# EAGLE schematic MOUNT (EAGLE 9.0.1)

## Sheet 1 of 2: Board to Board Headers
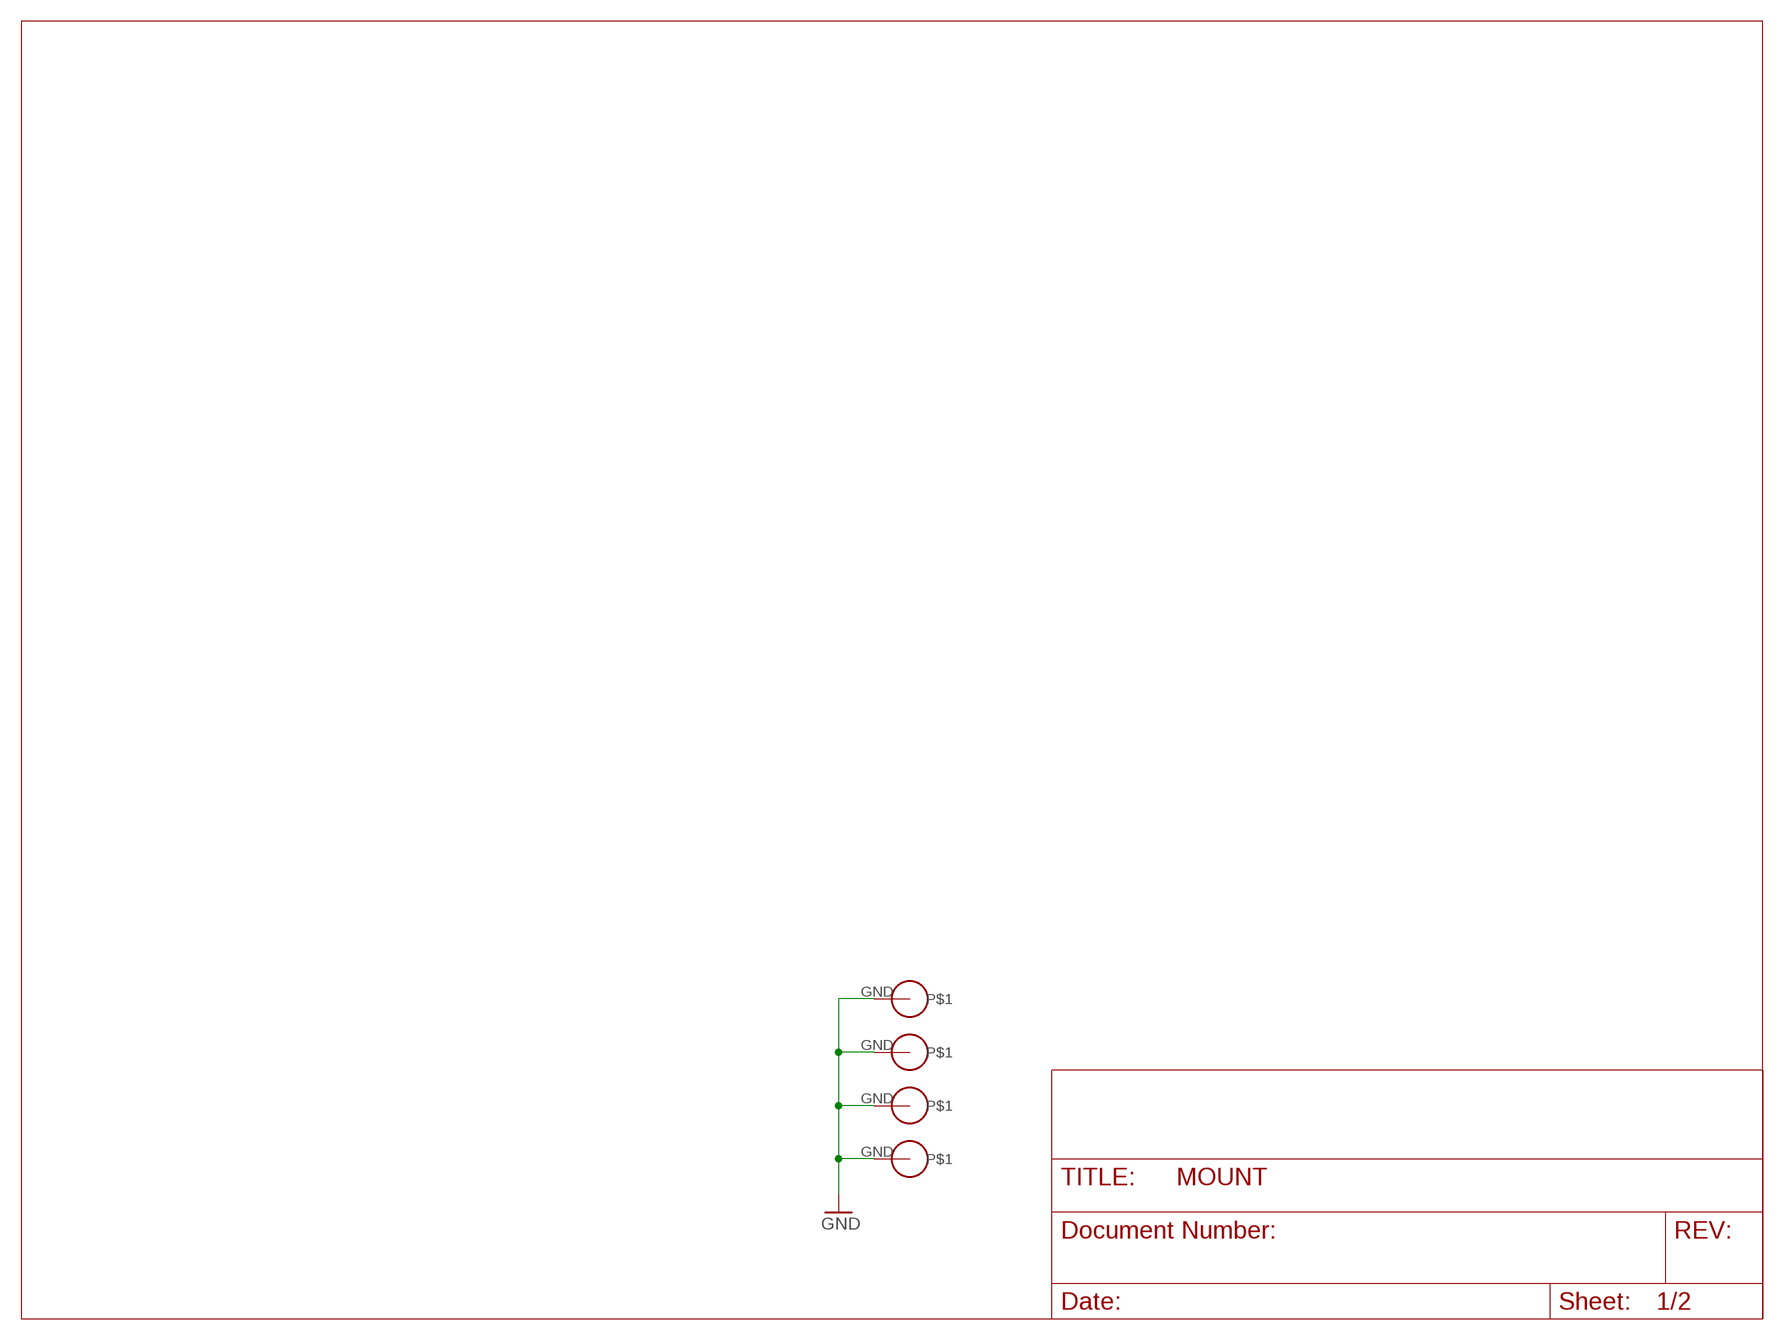
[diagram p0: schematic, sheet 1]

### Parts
U$1  PS/104-MOUNTING-HOLE  [PC/104-MOUNTING-HOLE]
U$2  PS/104-MOUNTING-HOLE  [PC/104-MOUNTING-HOLE]
U$3  PS/104-MOUNTING-HOLE  [PC/104-MOUNTING-HOLE]
U$4  PS/104-MOUNTING-HOLE  [PC/104-MOUNTING-HOLE]

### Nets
GND: U$1.GND U$2.GND U$3.GND U$4.GND

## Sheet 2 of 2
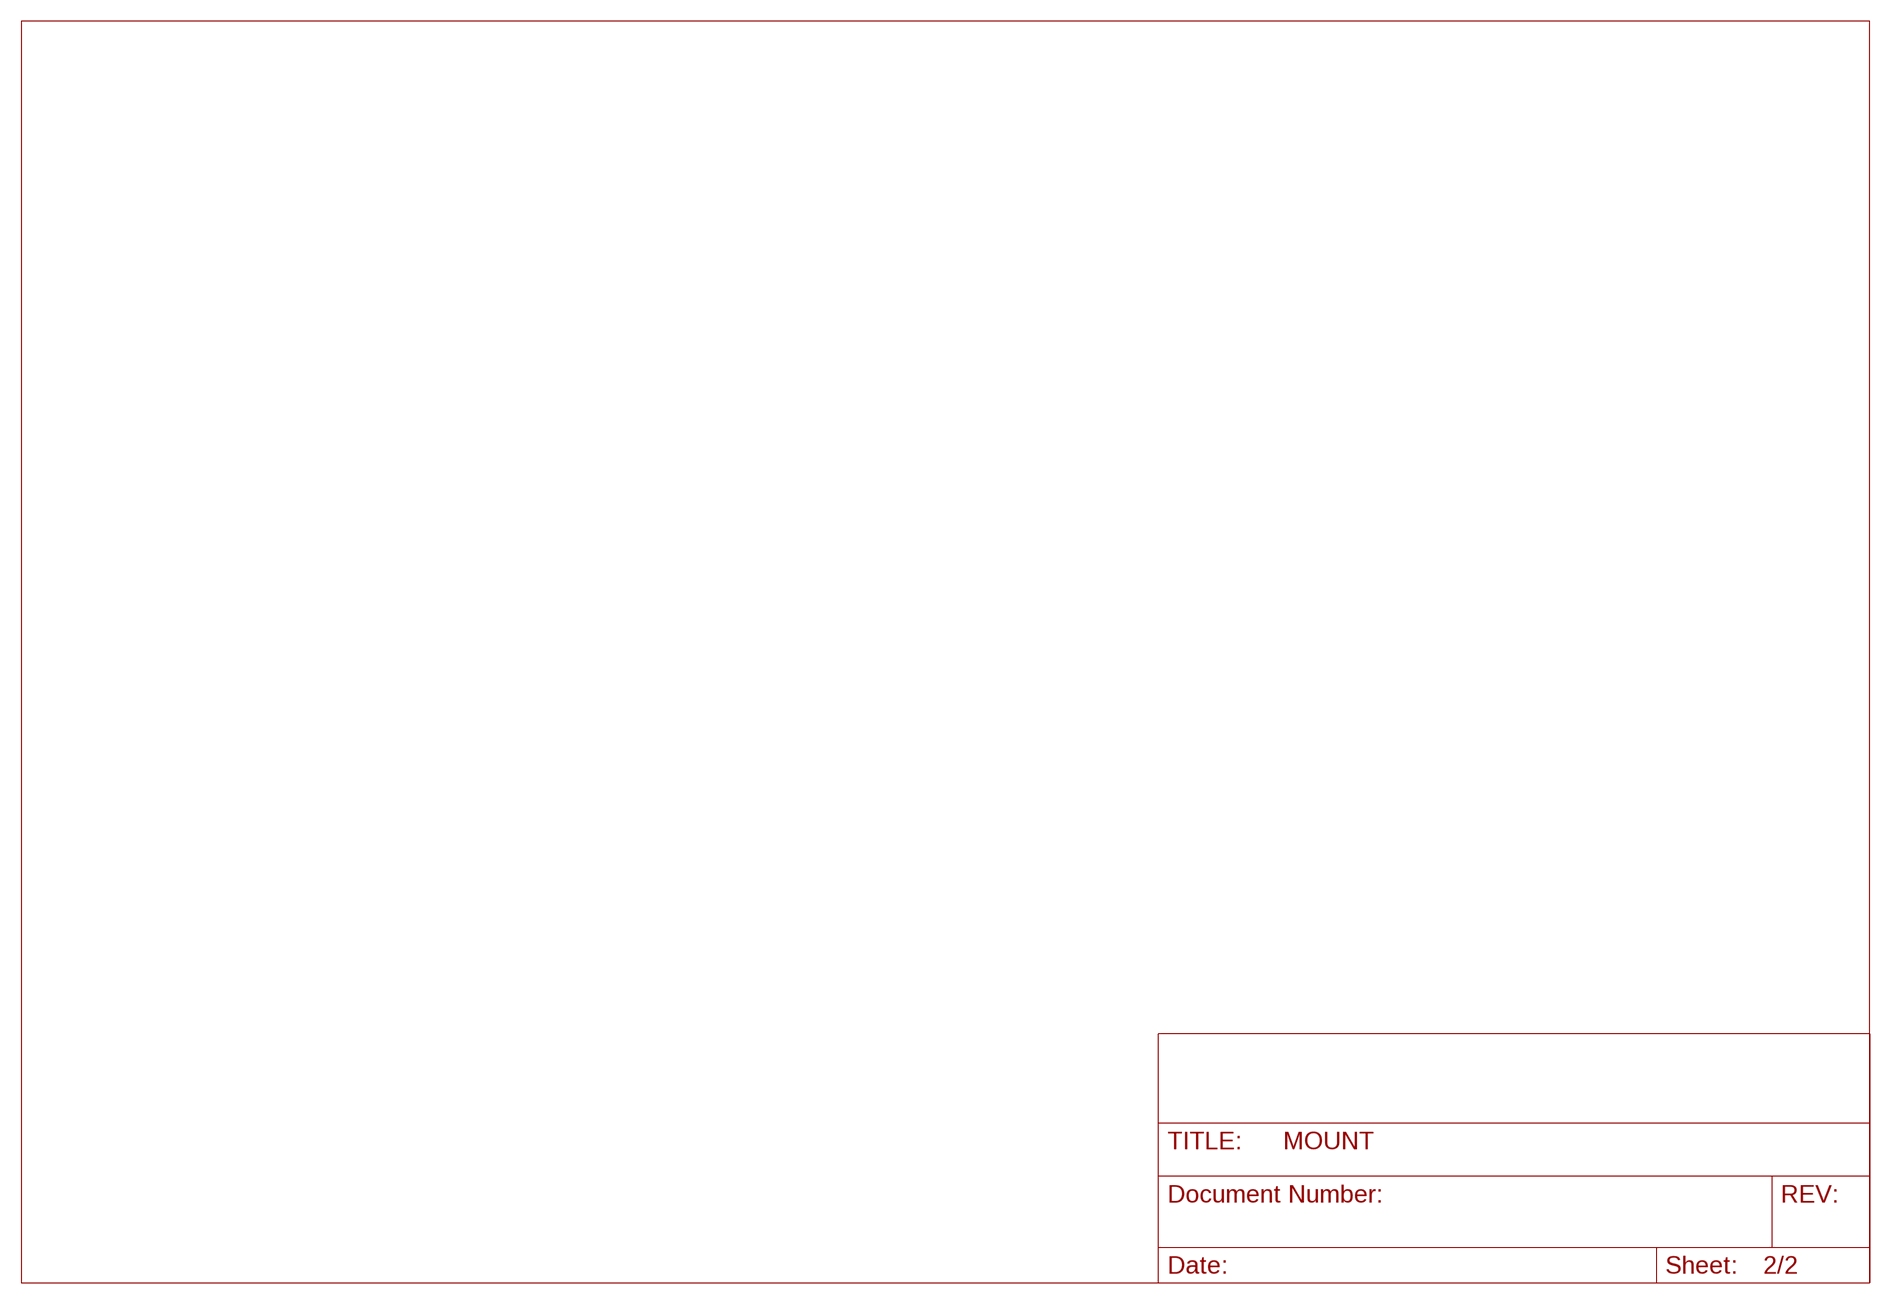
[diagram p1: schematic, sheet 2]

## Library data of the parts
U$1-U$4 = CU inSpace 2019 Parts:PS/104-MOUNTING-HOLE: Mounting hole for PC/104 board.

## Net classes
0 default: clearance 0.205 mm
